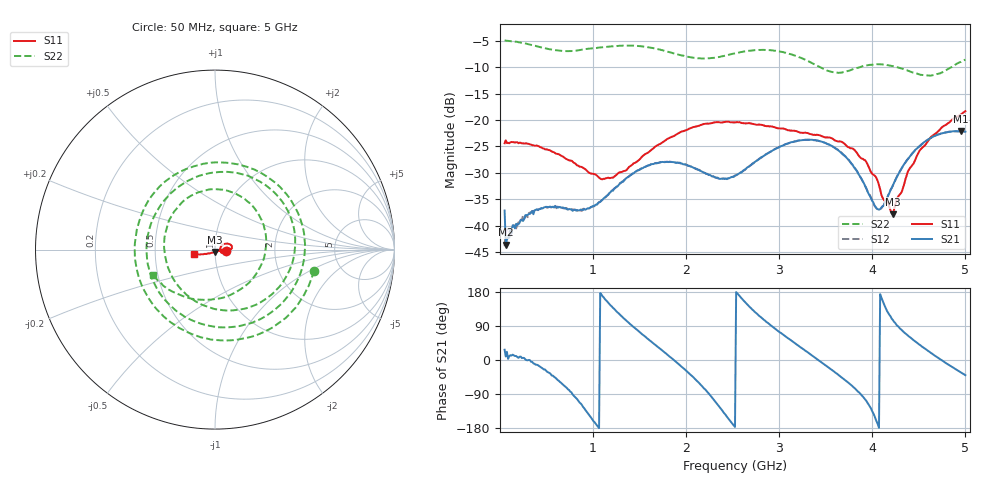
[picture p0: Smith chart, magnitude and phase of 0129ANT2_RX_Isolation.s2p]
! MASWSS0129 de-embedded Sparameters using port extention method. ANT2 to RX Isolation using 3 volt control
! 100pF blocking capacitor
! Sample board 1000013136
# Hz  S  DB  R  50
! Freq  S11  S21  S12  S22
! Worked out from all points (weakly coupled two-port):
!   401 points, 50 MHz to 5 GHz, reference 50 ohm
!   highest |S21| = -22.08 dB at 4.95 GHz (marker M1); lowest = -43.6 dB at 62.38 MHz (marker M2)
!   lowest |S11| = -37.8 dB at 4.22 GHz (marker M3), VSWR 1.03, Z = 50.1 - j1.28 ohm
!   |S11| at or under -10 dB: start of sweep to end of sweep
!   |S22| runs from -11.6 to -5.0 dB; largest |S21 - S12| = 0.011
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5e7  -24.39 -5.5  -37.11 27.1  -43.85 -21.8  -4.96 -12.0
6.2375e7  -23.84 -2.3  -43.57 9.2  -41.34 1.5  -5.00 -15.1
2.48e8  -24.38 -11.4  -39.09 5.8  -38.07 6.6  -5.45 -59.2
4.08875e8  -24.92 -17.4  -36.95 -13.9  -37.04 -15.0  -6.11 -99.0
6.44e8  -26.59 -24.7  -36.42 -57.7  -36.51 -56.4  -6.90 -159.9
8.79125e8  -28.88 -23.8  -36.96 -118.0  -37.18 -119.1  -6.71 141.0
1.12663e9  -31.12 -3.5  -34.63 160.8  -34.69 161.6  -6.21 80.5
1.3865e9  -28.88 24.1  -30.67 97.6  -30.63 97.4  -5.93 21.1
1.70825e9  -24.62 32.1  -28.08 32.1  -28.06 32.0  -6.66 -54.1
1.90625e9  -22.62 26.8  -28.04 -8.0  -28.05 -8.4  -7.60 -104.3
2.129e9  -21.11 19.6  -29.39 -58.0  -29.43 -58.4  -8.33 -164.7
2.525e9  -20.45 6.9  -30.52 -176.7  -30.50 -176.6  -7.40 94.3
2.95813e9  -21.42 2.6  -25.49 82.2  -25.44 81.9  -6.91 8.0
3.35413e9  -22.75 7.0  -23.74 11.6  -23.76 11.5  -9.26 -79.9
3.713e9  -24.69 6.5  -26.94 -54.1  -26.91 -54.2  -10.85 170.8
4.04713e9  -31.08 -15.7  -36.76 -162.6  -36.73 -161.4  -9.45 90.6
4.18325e9  -36.43 -58.1  -33.80 119.1  -33.84 118.7  -9.71 61.5
4.22038e9  -37.82 -86.8  -32.37 105.7  -32.41 105.3  -9.81 53.0
4.505e9  -25.90 -152.9  -24.97 40.7  -25.00 41.0  -11.38 -20.7
4.71538e9  -21.99 -161.3  -22.69 4.3  -22.70 4.1  -11.24 -87.0
4.9505e9  -18.96 -166.6  -22.08 -32.4  -22.18 -33.3  -9.04 -147.8
5e9  -18.33 -167.7  -22.21 -40.1  -22.23 -40.4  -8.59 -157.4
